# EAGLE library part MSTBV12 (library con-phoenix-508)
PHOENIX
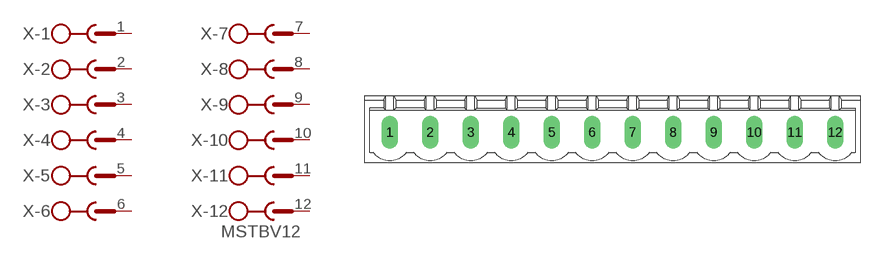
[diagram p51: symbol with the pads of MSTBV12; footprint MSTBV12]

Designator prefix X; gates -1=SK -2=SK -3=SK -4=SK -5=SK -6=SK -7=SK -8=SK -9=SK -10=SK -11=SK -12=SKV

## MSTBV12 (MPN: MSTBVA2.5/12-G-5.08; OC_FARNELL: 3705341; OC_NEWARK: 69K5694)  [MSTBV12]
1  -1:1  pas
2  -2:1  pas
3  -3:1  pas
4  -4:1  pas
5  -5:1  pas
6  -6:1  pas
7  -7:1  pas
8  -8:1  pas
9  -9:1  pas
10  -10:1  pas
11  -11:1  pas
12  -12:1  pas

## Footprint MSTBV12 (pad centres in mm)
PHOENIX
drill 1.397 long: 1 -27.94,0; 2 -22.86,0; 3 -17.78,0; 4 -12.7,0; 5 -7.62,0; 6 -2.54,0; 7 2.54,0; 8 7.62,0; 9 12.7,0; 10 17.78,0; 11 22.86,0; 12 27.94,0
